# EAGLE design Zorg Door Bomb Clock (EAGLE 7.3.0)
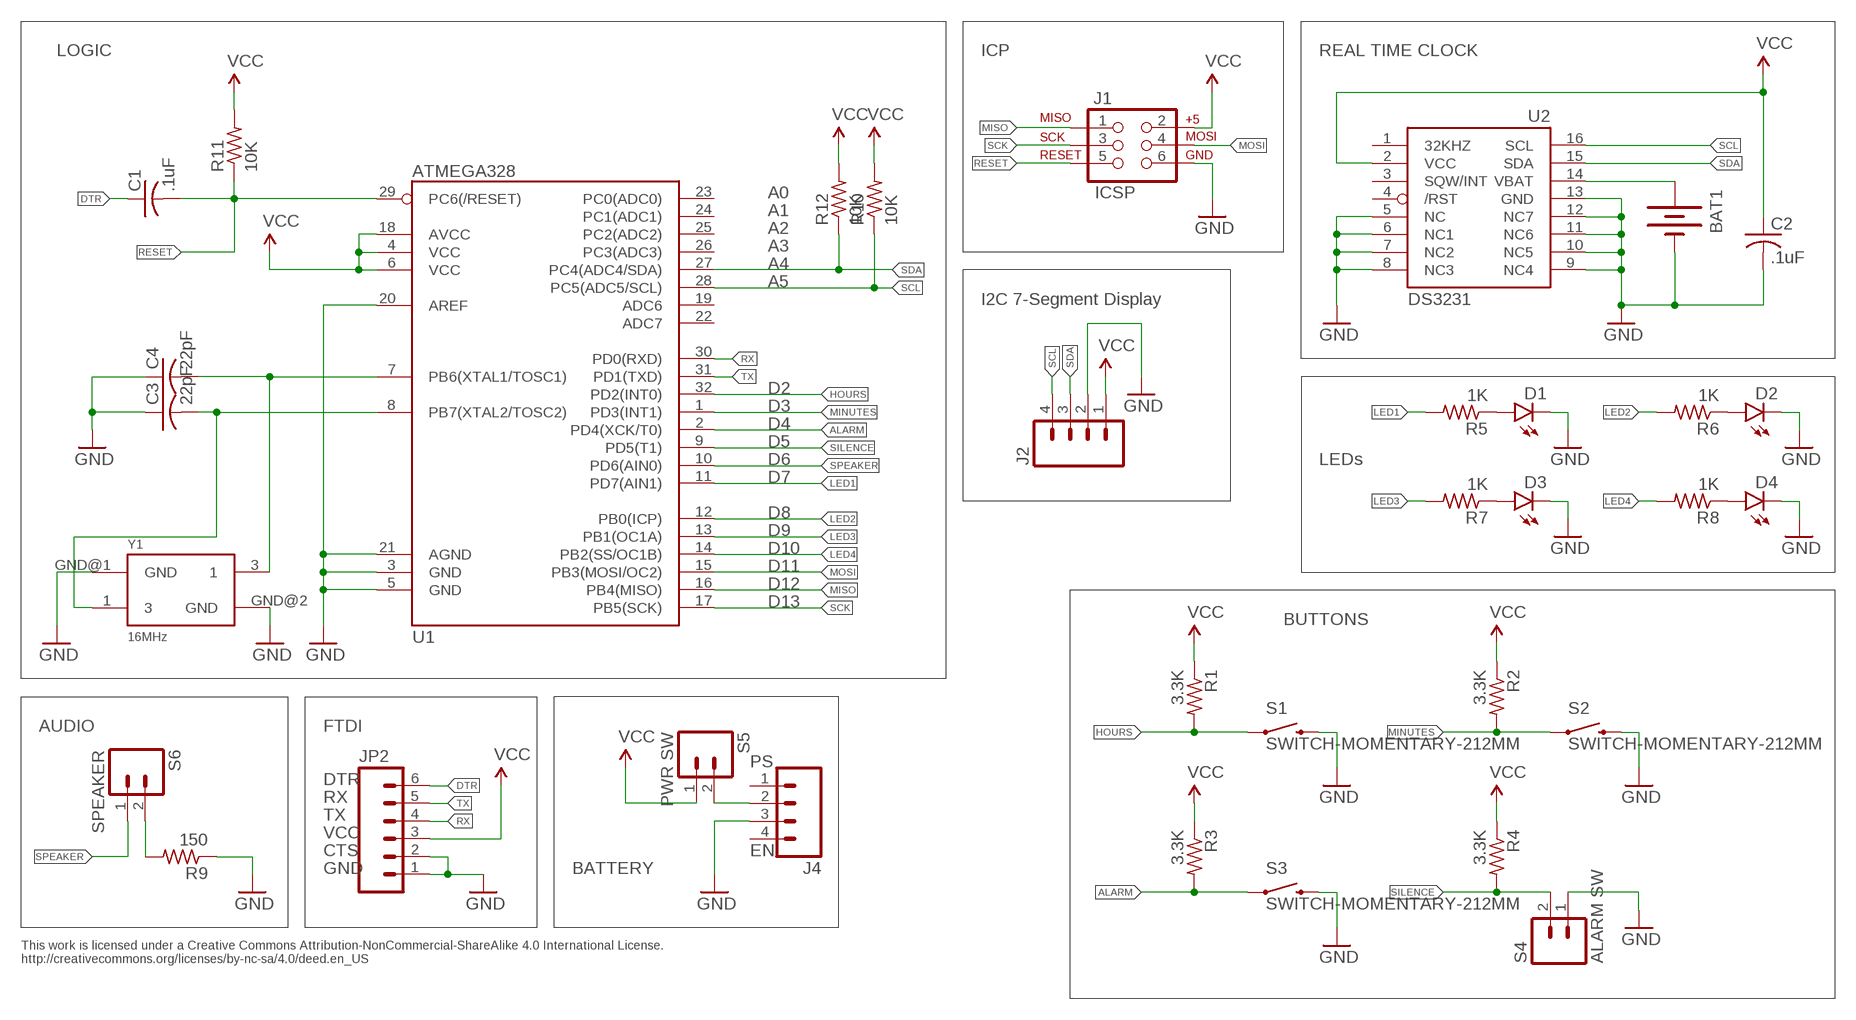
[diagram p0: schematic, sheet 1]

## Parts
BAT1  BATTERY12MM  [BATTCON_12MM]
C1  .1uF  C-USC0805K  [C0805K]
C2  .1uF  C-USC0805K  [C0805K]
C3  22pF  C-USC0805K  [C0805K]
C4  22pF  C-USC0805K  [C0805K]
D1  LED5MM  [LED5MM]
D2  LED5MM  [LED5MM]
D3  LED5MM  [LED5MM]
D4  LED5MM  [LED5MM]
J1  ICSP  AVR_SPI_PRG_6PTH  [2X3]
J2  M04NO_SILK_ALL_ROUND  [1X04_NO_SILK_ALL_ROUND]
J4  M04NO_SILK_ALL_ROUND  [1X04_NO_SILK_ALL_ROUND]
JP2  M06NO_SILK_FEMALE_PTH  [1X06_NO_SILK]
R1  3.3K  R-US_R0805  [R0805]
R2  3.3K  R-US_R0805  [R0805]
R3  3.3K  R-US_R0805  [R0805]
R4  3.3K  R-US_R0805  [R0805]
R5  1K  R-US_R0805  [R0805]
R6  1K  R-US_R0805  [R0805]
R7  1K  R-US_R0805  [R0805]
R8  1K  R-US_R0805  [R0805]
R9  150  R-US_R0805  [R0805]
R10  10K  R-US_R0805  [R0805]
R11  10K  R-US_R0805  [R0805]
R12  10K  R-US_R0805  [R0805]
S1  SWITCH-MOMENTARY-212MM  [TACTILE-PTH-12MM]
S2  SWITCH-MOMENTARY-212MM  [TACTILE-PTH-12MM]
S3  SWITCH-MOMENTARY-212MM  [TACTILE-PTH-12MM]
S4  ALARM SW  M02PTH  [1X02]
S5  PWR SW  M02PTH  [1X02]
S6  SPEAKER  M02PTH  [1X02]
U1  ATMEGA328  ATMEGA328_SMT  [TQFP32-08]
U2  DS3231  DS3231/SO  [SO16W]
Y1  16MHz  OSCILLATOR5X3  [CRYSTAL-SMD-5X3]

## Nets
ALARM: R3.2 S3.1 U1.2(PD4(XCK/T0))
DTR: C1.1 JP2.6
GND: BAT1.GND(-) C2.2 C3.1 C4.1 D1.K(C) D2.K(C) D3.K(C) D4.K(C) J1.6 J2.2 J4.3 JP2.1 JP2.2 R9.1 S1.3 S2.3 S3.3 S4.1 U1.3(GND) U1.5(GND) U1.20(AREF) U1.21(AGND) U2.5(NC) U2.6(NC1) U2.7(NC2) U2.8(NC3) U2.9(NC4) U2.10(NC5) U2.11(NC6) U2.12(NC7) U2.13(GND) Y1.GND@1(GND) Y1.GND@2(GND)
HOURS: R1.2 S1.1 U1.32(PD2(INT0))
LED1: R5.2 U1.11(PD7(AIN1))
LED2: R6.2 U1.12(PB0(ICP))
LED3: R7.2 U1.13(PB1(OC1A))
LED4: R8.2 U1.14(PB2(SS/OC1B))
MINUTES: R2.2 S2.1 U1.1(PD3(INT1))
MISO: J1.1 U1.16(PB4(MISO))
MOSI: J1.4 U1.15(PB3(MOSI/OC2))
N$1: D1.A R5.1
N$2: D4.A R8.1
N$3: D3.A R7.1
N$4: D2.A R6.1
N$5: J4.2 S5.2
N$8: C3.2 U1.8(PB7(XTAL2/TOSC2)) Y1.1
N$10: C4.2 U1.7(PB6(XTAL1/TOSC1)) Y1.3
N$15: BAT1.PWR@1(+) U2.14(VBAT)
N$16: R9.2 S6.2
RESET: C1.2 J1.5 R11.1 U1.29(PC6(/RESET))
RX: JP2.4 U1.30(PD0(RXD))
SCK: J1.3 U1.17(PB5(SCK))
SCL: J2.4 R10.1 U1.28(PC5(ADC5/SCL)) U2.16(SCL)
SDA: J2.3 R12.1 U1.27(PC4(ADC4/SDA)) U2.15(SDA)
SILENCE: R4.2 S4.2 U1.9(PD5(T1))
SPEAKER: S6.1 U1.10(PD6(AIN0))
TX: JP2.5 U1.31(PD1(TXD))
VCC: C2.1 J1.2 J2.1 JP2.3 R1.1 R2.1 R3.1 R4.1 R10.2 R11.2 R12.2 S5.1 U1.4(VCC) U1.6(VCC) U1.18(AVCC) U2.2(VCC)
Unconnected: J4.1 J4.4 U1.19(ADC6) U1.22(ADC7) U1.23(PC0(ADC0)) U1.24(PC1(ADC1)) U1.25(PC2(ADC2)) U1.26(PC3(ADC3)) U2.1(32KHZ) U2.3(SQW/INT) U2.4(/RST)

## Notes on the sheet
- LOGIC | ICP | REAL TIME CLOCK
- A0
- A1
- A2
- A3
- A4
- A5
- I2C 7-Segment Display
- D2
- D3
- D4
- D5
- D6 | LEDs
- D7
- D8
- D9
- D10
- D11
- D12
- D13
- BUTTONS
- AUDIO | FTDI
- PS
- DTR
- RX
- TX
- VCC
- CTS | EN
- GND | BATTERY
- This work is licensed under a Creative Commons Attribution-NonCommercial-ShareAlike 4.0 International License.
  http://creativecommons.org/licenses/by-nc-sa/4.0/deed.en_US

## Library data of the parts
BAT1 = SparkFun-Electromechanical:BATTERY: Battery Holders; PROD_ID: BATT-08044
C1-C4 = adafruit:C-US: CAPACITOR, American symbol
D1-D4 = SparkFun-LED:LED: LEDs
J1 = SparkFun:AVR_SPI_PRG_6: AVR ISP 6 Pin This is the reduced ISP connector for AVR programming. Common on Arduino. This footprint will take up less PCB space and can be used with a 10-pin to 6-pin adapter such as SKU: BOB-08508; OC_NEWARK: unknown
J2 J4 = SparkFun-Connectors:M04: Header 4 Standard 4-pin 0.1" header. Use with straight break away headers (SKU : PRT-00116), right angle break away headers (PRT-00553), swiss pins (PRT-00743), machine pins (PRT-00117), and female headers (PRT-00115). Molex polarized connector foot print use with SKU : PRT-08231 with associated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; PROD_ID: CONN-09696
JP2 = SparkFun-Connectors:M06: Header 6 Standard 6-pin 0.1" header. Use with straight break away headers (SKU : PRT-00116), right angle break away headers (PRT-00553), swiss pins (PRT-00743), machine pins (PRT-00117), and female headers (PRT-00115). Molex polarized connector foot print use with SKU : PRT-08094 with associated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; PROD_ID: CONN-08437
R1-R12 = adafruit:R-US_: RESISTOR, American symbol
S1-S3 = SparkFun-Electromechanical:SWITCH-MOMENTARY-2: Various NO switches- pushbuttons, reed, etc; PROD_ID: SWCH-09185
S4-S6 = SparkFun-Connectors:M02: Standard 2-pin 0.1" header. Use with
U1 = SparkFun-DigitalIC:ATMEGA328_SMT: 32-Pin Atmega328 part Commonly used on Arduino compatible boards Available in QFP and QFN packages TQFP is IC-09069 QFN is non-stock; PROD_ID: IC-09069; VALUE: ATMEGA328P
U2 = adafruit:DS3231
Y1 = SparkFun-FreqCtrl:OSCILLATOR: Generic 5x3 and 7x5 oscillators

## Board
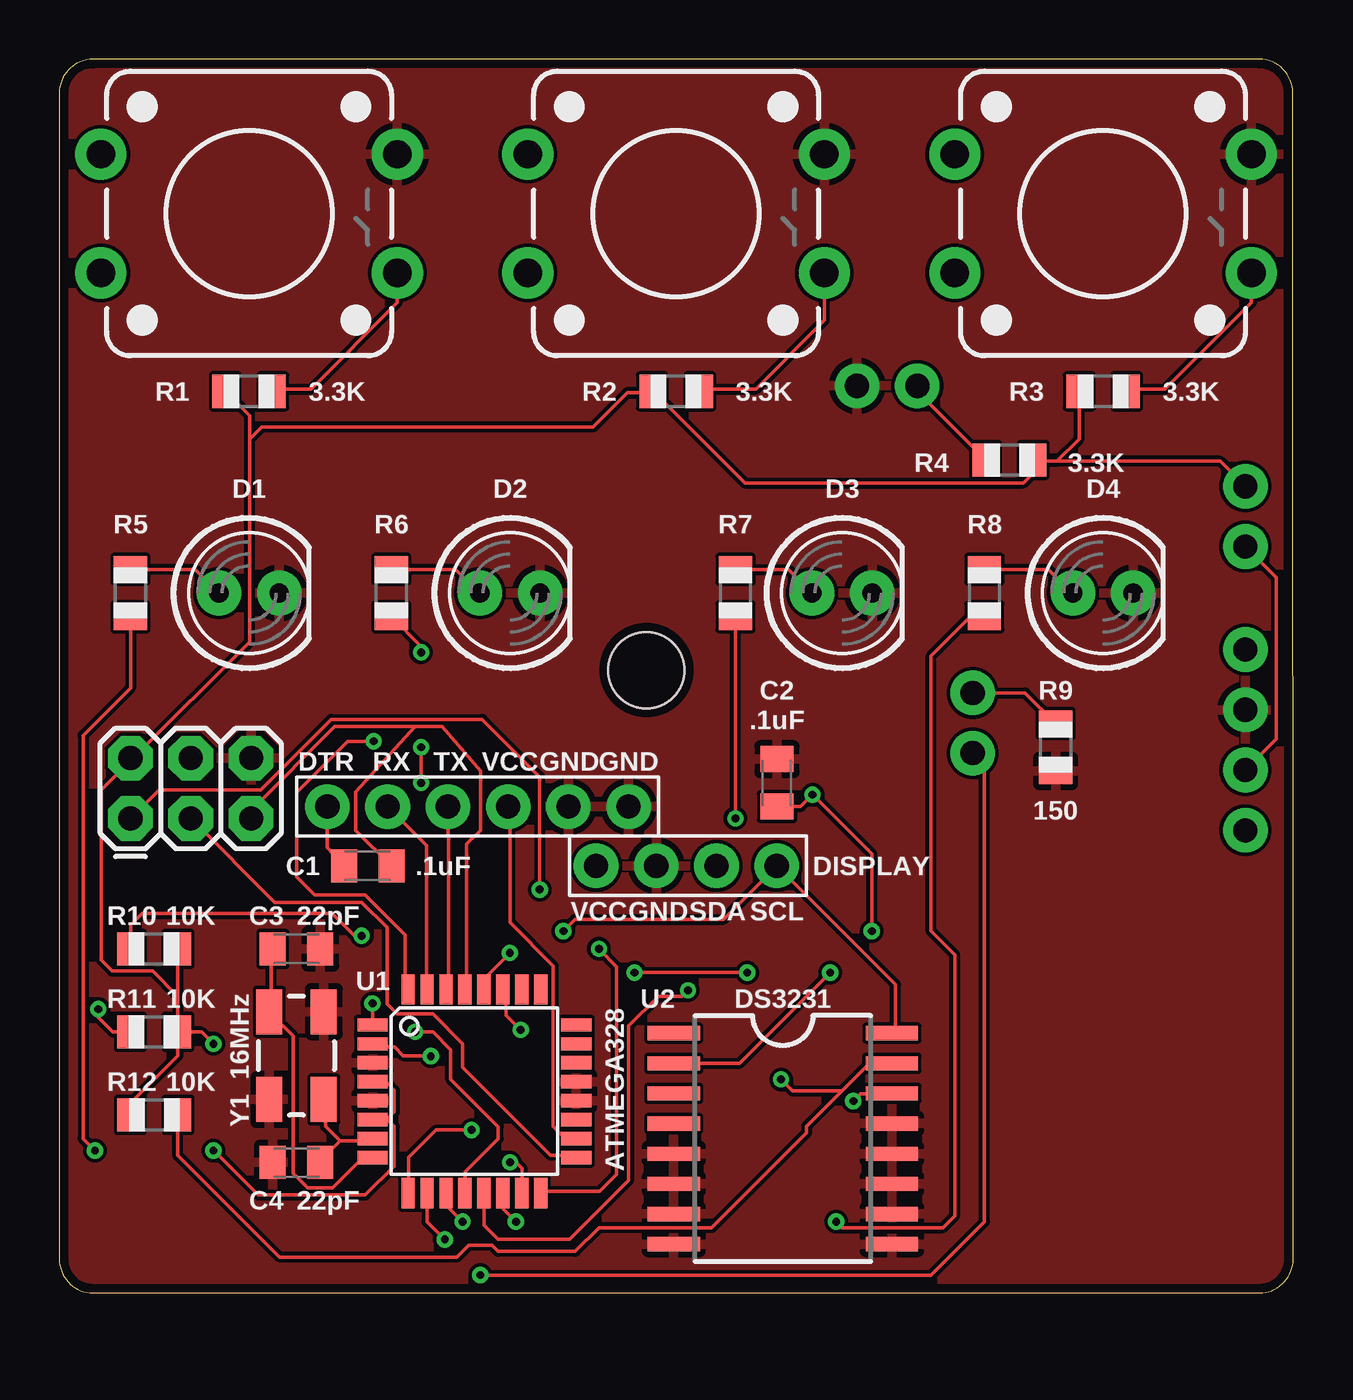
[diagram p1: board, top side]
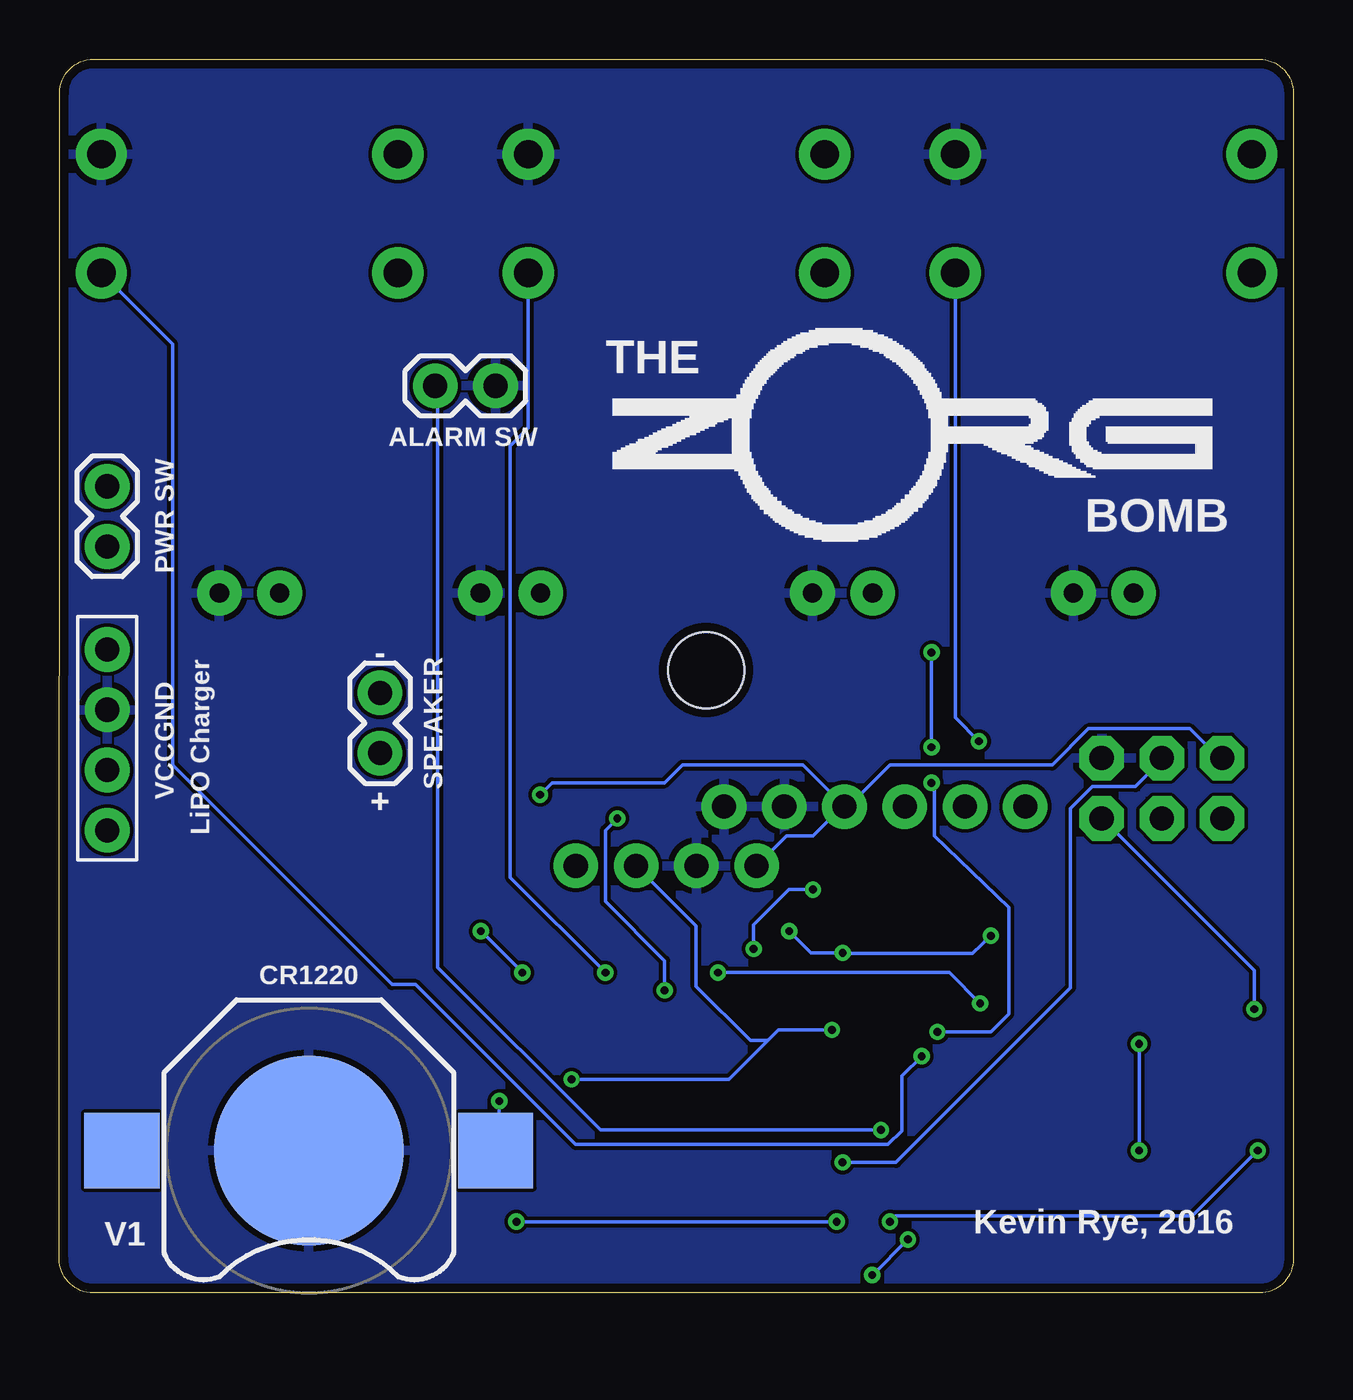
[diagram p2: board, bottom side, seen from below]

Size 52.02 x 52 mm. Coordinates in mm from the lower left corner, seen from the top.
Outline: 1.41,0 50.59,0 arc90 52.02,1.43 52,50.59 arc90 50.59,52 1.41,52 arc90 0,50.59 0,1.41 arc90 1.41,0
Copper layers (1*16): Top 0.0356mm / dielectric 1.5011mm / Bottom 0.0356mm
Design rules "LaenPCBOrder": minimum track width 6mil, minimum drill 13mil, track to track 6mil, track to pad 6mil, pad to pad 6mil, via to via 6mil, smd to smd 6mil, copper to edge 15mil, drill to drill 6mil, minimum pad ring 7mil, minimum via ring 7mil, stop-mask expansion 3mil, vias tented up to drill 0mil, thermal gap 10mil
Holes 3.2 mm at 24.75,26.25

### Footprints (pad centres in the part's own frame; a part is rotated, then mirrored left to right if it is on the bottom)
BATTCON_12MM = smd 8 x 8: GND 0,0 | smd 3.175 x 3.175: PWR@1 -7.874,0; PWR@2 7.874,0
C0805K = smd 1.1 x 1.4: 1 -1,0; 2 1,0
LED5MM = drill 0.813 pad 1.88: A -1.27,0; K 1.27,0
2X3 = drill 1.016 pad 1.88 octagon: 1 0,0; 2 0,2.54; 3 2.54,0; 4 2.54,2.54; 5 5.08,0; 6 5.08,2.54
1X04_NO_SILK_ALL_ROUND = drill 1.016 pad 1.88: 1 0,0; 2 2.54,0; 3 5.08,0; 4 7.62,0
1X06_NO_SILK = drill 1.016 pad 1.88: 1 0,0; 2 2.54,0; 3 5.08,0; 4 7.62,0; 5 10.16,0; 6 12.7,0
R0805 = smd 1.1 x 1.4: 1 -1,0; 2 1,0
TACTILE-PTH-12MM = drill 1.2 pad 2.159: 1 6.25,-2.5; 2 -6.25,-2.5; 3 6.25,2.5; 4 -6.25,2.5
1X02 = drill 1.016 pad 1.88: 1 0,0; 2 2.54,0
TQFP32-08 = smd 1.27 x 0.559: 1 -4.293,2.8; 2 -4.293,2; 3 -4.293,1.2; 4 -4.293,0.4; 5 -4.293,-0.4; 6 -4.293,-1.2; 7 -4.293,-2; 8 -4.293,-2.8; 17 4.293,-2.8; 18 4.293,-2; 19 4.293,-1.2; 20 4.293,-0.4; 21 4.293,0.4; 22 4.293,1.2; 23 4.293,2; 24 4.293,2.8 | smd 0.559 x 1.27: 9 -2.8,-4.293; 10 -2,-4.293; 11 -1.2,-4.293; 12 -0.4,-4.293; 13 0.4,-4.293; 14 1.2,-4.293; 15 2,-4.293; 16 2.8,-4.293; 25 2.8,4.293; 26 2,4.293; 27 1.2,4.293; 28 0.4,4.293; 29 -0.4,4.293; 30 -1.2,4.293; 31 -2,4.293; 32 -2.8,4.293
SO16W = smd 0.6 x 2.2: 1 -4.445,-4.6; 2 -3.175,-4.6; 3 -1.905,-4.6; 4 -0.635,-4.6; 5 0.635,-4.6; 6 1.905,-4.6; 7 3.175,-4.6; 8 4.445,-4.6; 9 4.445,4.6; 10 3.175,4.6; 11 1.905,4.6; 12 0.635,4.6; 13 -0.635,4.6; 14 -1.905,4.6; 15 -3.175,4.6; 16 -4.445,4.6
CRYSTAL-SMD-5X3 = smd 1.9 x 1.1: 1 -1.85,-1.15; 3 1.85,1.15; GND@1 -1.85,1.15; GND@2 1.85,-1.15

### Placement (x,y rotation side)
BAT1  41.5,6 180 bottom
C1  13,18 0 top
C2  30.25,21.5 90 top
C3  10,14.5 180 top
C4  10,5.5 0 top
D1  8,29.5 0 top
D2  19,29.5 0 top
D3  33,29.5 0 top
D4  44,29.5 0 top
J1  3,20 0 top
J2  22.62,18 0 top
J4  50,19.5 90 bottom
JP2  24,20.5 180 top
R1  8,38 0 top
R2  26,38 0 top
R3  44,38 0 top
R4  40.05,35.11 180 top
R5  3,29.5 270 top
R6  14,29.5 270 top
R7  28.5,29.5 270 top
R8  39,29.5 270 top
R9  42,23 90 top
R10  4,14.5 0 top
R11  4,11 0 top
R12  4,7.5 180 top
S1  8,45.5 0 top
S2  26,45.5 0 top
S3  44,45.5 0 top
S4  33.63,38.23 180 bottom
S5  50,34 270 bottom
S6  38.5,22.75 90 bottom
U1  17.5,8.5 0 top
U2  30.5,6.5 270 top
Y1  10,10 270 top

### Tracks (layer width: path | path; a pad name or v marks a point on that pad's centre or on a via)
ALARM  (via drill 0.33)
  Top 0.152: U1.2 13.36,10.37 14.13,10.37 14.5,10 15.64,10 v15.66,9.97 | R3.2 45.05,38.11 46.61,38.11 50.25,41.75 S3.1
  Bottom 0.152: 50.24,42.98 S3.1 47.25,40 47.25,22.25 38,13 37,13 30.26,6.26 17.08,6.26 16.5,6.83 16.5,9.14 v15.66,9.97
DTR
  Top 0.152: C1.1 11.3,18.79 JP2.6
GND
  pour Top: -2,53 55,53 55,-1 -2,-1
  pour Bottom: -1.25,52.5 53.75,52.5 54,-0.5 -1,-0.5
HOURS  (via drill 0.33)
  Top 0.152: U1.32 14.57,12.81 14.57,15.1 12.9,16.77 10.76,16.77 10,17.53 10,21.09 12.16,23.25 v13.25,23.25 | R1.2 9.09,38.11 10.61,38.11 14.25,41.75 S1.1
  Bottom 0.152: 14.12,42.98 S1.1 14.25,24.25 v13.25,23.25
LED1  (via drill 0.33)
  Top 0.152: R5.2 3,25.5 1,23.5 1,6.5 v1.5,6 | v17,3 16.3,3.7 U1.11
  Bottom 0.152: v17,3 16.75,3.25 4.25,3.25 v1.5,6
LED2  (via drill 0.33)
  Top 0.152: U1.12 17.1,5.1 18.5,6.5 18.5,7 16.5,9 16.5,10.25 15.75,11 v15,11 | v15.25,21.5 v15.25,23 | v15.25,27 15.25,27.25 R6.2
  Bottom 0.152: v15,11 12.75,11 12,11.75 12,16.25 15.12,19.25 15.12,21.25 v15.25,21.5 | v15.25,23 v15.25,27
LED3  (via drill 0.33)
  Top 0.152: U1.13 17.9,2.85 18.5,2.25 21.5,2.25 24,4.75 24,11.25 25.25,12.5 26.25,12.5 v26.5,12.75 | 28,28.5 R7.2 28.5,21 v28.5,20
  Bottom 0.152: v26.5,12.75 26.5,14 29,16.5 29,19.5 v28.5,20
LED4  (via drill 0.33)
  Top 0.152: v19.25,3 18.7,3.55 U1.14 | v32.75,3 33,2.75 37.25,2.75 37.75,3.25 37.75,14.25 36.75,15.25 36.75,26.84 38.41,28.5 R8.2
  Bottom 0.152: v32.75,3 v19.25,3
MINUTES  (via drill 0.33)
  Top 0.152: v13.2,12.2 13.2,11.44 U1.1 | R2.2 27.07,38.11 29.36,38.11 32.25,41 S2.1 | v24.25,13.5 v29,13.5
  Bottom 0.152: S2.1 32.25,42.98 32.25,36.45 33.01,35.69 33.01,17.51 v29,13.5 | v24.25,13.5 14.5,13.5 v13.2,12.2
MISO  (via drill 0.33)
  Top 0.152: U1.16 20.36,4.27 22.77,4.27 23.5,5 23.5,13.75 v22.75,14.5 | J1.1 3.14,20.12 4.21,21.19 8.48,21.19 11.46,24.17 17.83,24.17 20.25,21.75 v20.25,17
  Bottom 0.152: v20.25,17 21.25,17 22.75,15.5 v22.75,14.5
MOSI  (via drill 0.33)
  Top 0.152: 19.45,4.27 U1.15 19.5,5.25 19.25,5.5 v19,5.5
  Bottom 0.152: J1.4 5.58,22.41 6.65,21.34 8.48,21.34 9.39,20.43 9.39,12.86 16.75,5.5 v19,5.5
N$1
  Top 0.152: R5.1 3.14,30.49 5.74,30.49 6.65,29.57 D1.A
N$2
  Top 0.152: R8.1 39.11,30.49 41.7,30.49 42.62,29.57 D4.A
N$3
  Top 0.152: D3.A 31.64,29.57 30.73,30.49 28.14,30.49 28.15,30.5 R7.1
N$4
  Top 0.152: R6.1 14.12,30.49 16.71,30.49 17.62,29.57 D2.A
N$5
  Top 0.152: J4.2 51.3,23.34 51.3,30.16 S5.2
N$8
  Top 0.152: U1.8 13.2,5.65 12.74,5.65 11.53,4.43 10.46,4.43 9.85,5.04 9.85,10.83 8.94,11.74 Y1.1 8.94,11.89 8.94,14.48 C3.2
N$10
  Top 0.152: 11.83,6.41 13.2,6.41 U1.7 | 11.83,6.41 11.07,5.65 C4.2 | 11.83,6.41 11.22,7.02 11.22,8.08 Y1.3
N$15  (via drill 0.33)
  Top 0.152: v33.47,8.08 33.78,8.39 35,8.39 U2.14
  Bottom 0.152: v33.47,8.08 33.47,6.26 33.62,6.1 BAT1.PWR@1
N$16
  Top 0.152: S6.2 40.71,25.29 R9.2
RESET  (via drill 0.33)
  Top 0.152: U1.29 17.16,12.81 17.16,18.91 17.75,19.5 17.75,22 16.13,23.87 15,23.87 | 3.14,11.13 R11.1 2.26,11 1.64,11.61 v1.64,11.96 | J1.5 8.17,20.12 8.17,20.43 11.61,23.87 15,23.87 | 15,23.87 12.5,21.12 12.5,19.5 C1.2
  Bottom 0.152: v1.64,11.96 1.64,13.6 8.02,19.97 J1.5
RX
  Top 0.152: U1.30 16.4,12.81 16.4,17.99 JP2.4
SCK
  Top 0.152: U1.17 21.74,5.8 20.7,5.8 17,9.5 17,10.5 15.75,11.75 14.25,11.75 13.81,12.19 13.81,15.4 12.74,16.47 9.09,16.47 5.58,19.97 J1.3
SCL  (via drill 0.33)
  Top 0.152: v18.99,14.33 17.93,13.27 17.93,12.81 U1.28 | 3.45,14.64 3.14,14.64 R10.1 3,15.5 3.5,16 11.5,16 12.45,15.05 v12.74,15.05 | 35.15,10.98 U2.16 35.25,11.1 35.25,12.99 J2.4 28,15.75 21.75,15.75 v21.25,15.25
  Bottom 0.152: v12.74,15.05 13.52,14.3 18.96,14.3 arc90 v18.99,14.33 | 18.99,14.36 v18.99,14.33 | v18.99,14.33 20.33,14.33 v21.25,15.25
SDA  (via drill 0.33)
  Top 0.152: U1.27 18.84,12.66 18.84,11.7 v19.45,11.09 | 32.99,8.51 34.08,9.61 35,9.61 U2.15 | 32.99,8.51 31.5,7.03 31.5,6.75 27.5,2.75 22.75,2.75 21.75,1.75 18.5,1.75 18.25,2 17.25,2 16.75,1.5 9.29,1.5 5,5.79 R12.1 | v30.42,9 30.91,8.51 32.99,8.51
  Bottom 0.152: v19.45,11.09 21.69,11.09 22.14,10.64 | 22.14,10.64 23.79,9 v30.42,9 | 22.14,10.64 22.89,10.64 25.17,12.92 25.17,15.46 J2.3
SILENCE  (via drill 0.33)
  Top 0.152: U1.9 14.73,4.27 14.73,5.71 15.89,6.87 v17.38,6.87 | R4.2 38.96,35.21 36.06,38.11 S4.2
  Bottom 0.152: v17.38,6.87 29.2,6.87 36.06,13.72 36.06,38.11 S4.2
SPEAKER  (via drill 0.33)
  Top 0.152: U1.10 15.64,4.12 arc90 15.5,3.98 15.5,3 v16.25,2.25 | v17.75,0.75 36.75,0.75 39,3 39,22.25 S6.1
  Bottom 0.152: v16.25,2.25 v17.75,0.75
TX
  Top 0.152: U1.31 15.49,12.81 15.49,18.85 JP2.5
VCC  (via drill 0.33)
  Top 0.152: U1.18 21.74,6.56 21.28,6.56 20.82,7.02 20.82,13.78 18.99,15.61 18.99,20.5 JP2.3 | 41.09,35.21 R4.1 | 42.92,37.95 R3.1 | 43.38,37.95 43.07,37.95 R3.1 | 13.81,7.32 13.36,7.32 U1.6 13.81,7.32 | 13.81,7.32 14.12,7.63 14.12,8.54 13.81,8.85 13.36,8.85 U1.4 | 4.97,10.98 R11.2 | 4.97,14.48 R10.2 5,12.5 | 4.97,11.13 R11.2 | 13.81,7.32 14.12,7.02 14.12,5.34 12.9,4.12 8.38,4.12 v6.5,6 | 7.11,37.95 R1.1 8.02,36.98 8.02,36 | 40.63,35.06 40.94,35.06 | 40.94,35.06 R4.1 | R11.2 5,10 3,8 R12.2 | v6.5,10.5 6,11 R11.2 | 40.94,35.06 42.06,35.06 | 42.06,35.06 43,36 R3.1 | R4.1 41,35.06 41,34.5 40.65,34.15 28.9,34.15 25.09,37.95 R2.1 24.94,37.95 23.95,37.95 22.5,36.5 8.52,36.5 8.02,36 | 42.06,35.06 48.94,35.06 S5.1 | 8.02,36 8.02,27.44 3.14,22.56 J1.2 2.99,22.41 1.77,21.19 1.77,14.03 2.23,13.57 3.93,13.57 5,12.5 | 26.72,9.5 26.46,9.76 26,9.76 U2.2 28.68,9.68 v32.5,13.5 | 5,12.5 R11.2 | C2.1 31.25,20.5 v31.75,21 34.25,18.5 v34.25,15.25
  Bottom 0.152: J1.2 3.14,22.56 4.36,23.78 8.63,23.78 10.16,22.25 17,22.25 18.75,20.5 JP2.3 | v6.5,6 v6.5,10.5 | JP2.3 19,20.5 20.25,19.25 21.38,19.25 J2.1 | v31.75,21 31.25,21.5 26.5,21.5 25.75,22.25 20.67,22.25 JP2.3 | v32.5,13.5 v34.25,15.25

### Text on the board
Unrouted: This work is licensed under a Creative Commons Attribution-NonCommercial-ShareAlike 4.0 International License. / http://creativecommons.org/licenses/by-nc-sa/4.0/deed.en_US
tNames: DTR | RX | TX | VCC | GND | GND | DISPLAY | VCC | GND | SDA | SCL
bNames: THE | BOMB | - | GND | LiPO Charger | VCC | + | CR1220 | Kevin Rye, 2016 | V1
